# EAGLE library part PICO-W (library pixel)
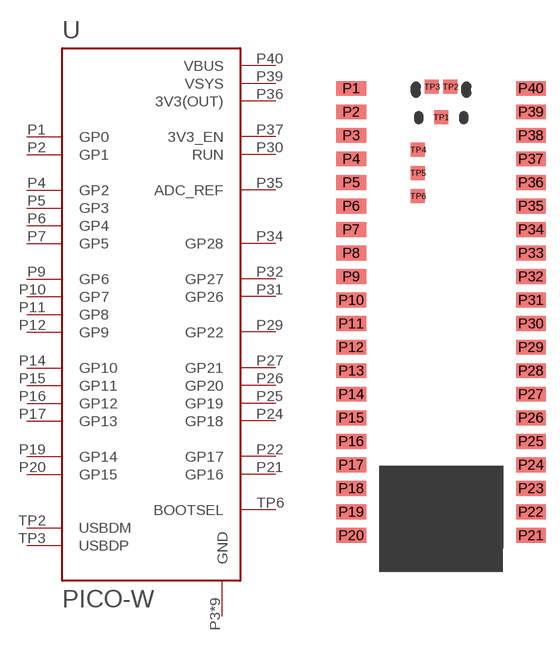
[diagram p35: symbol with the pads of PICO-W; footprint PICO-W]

Designator prefix -

## PICO-W  [PICO-W]
P1  GP0
P2  GP1
P3  GND  pwr
P4  GP2
P5  GP3
P6  GP4
P7  GP5
P8  GND  pwr
P9  GP6
P10  GP7
P11  GP8
P12  GP9
P13  GND  pwr
P14  GP10
P15  GP11
P16  GP12
P17  GP13
P18  GND  pwr
P19  GP14
P20  GP15
P21  GP16
P22  GP17
P23  GND  pwr
P24  GP18
P25  GP19
P26  GP20
P27  GP21
P28  GND  pwr
P29  GP22
P30  RUN  in
P31  GP26
P32  GP27
P33  GND  pwr
P34  GP28
P35  ADC_REF  in
P36  3V3(OUT)  pwr
P37  3V3_EN  in
P38  GND  pwr
P39  VSYS  pwr
P40  VBUS  pwr
TP1  GND  pwr
TP2  USBDM  pwr
TP3  USBDP  pwr
TP6  BOOTSEL  pwr

## Footprint PICO-W (pad centres in mm)
smd 3.2 x 1.6: P1 0.81,49.63; P2 0.81,47.09; P3 0.81,44.55; P4 0.81,42.01; P5 0.81,39.47; P6 0.81,36.93; P7 0.81,34.39; P8 0.81,31.85; P9 0.81,29.31; P10 0.81,26.77; P11 0.81,24.23; P12 0.81,21.69; P13 0.81,19.15; P14 0.81,16.61; P15 0.81,14.07; P16 0.81,11.53; P17 0.81,8.99; P18 0.81,6.45; P19 0.81,3.91; P20 0.81,1.37; P21 20.19,1.37; P22 20.19,3.91; P23 20.19,6.45; P24 20.19,8.99; P25 20.19,11.53; P26 20.19,14.07; P27 20.19,16.61; P28 20.19,19.15; P29 20.19,21.69; P30 20.19,24.23; P31 20.19,26.77; P32 20.19,29.31; P33 20.19,31.85; P34 20.19,34.39; P35 20.19,36.93; P36 20.19,39.47; P37 20.19,42.01; P38 20.19,44.55; P39 20.19,47.09; P40 20.19,49.63
smd 1.5 x 1.5: TP1 10.5,46.5; TP2 11.5,49.8; TP3 9.5,49.8; TP4 8,43; TP5 8,40.5; TP6 8,38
